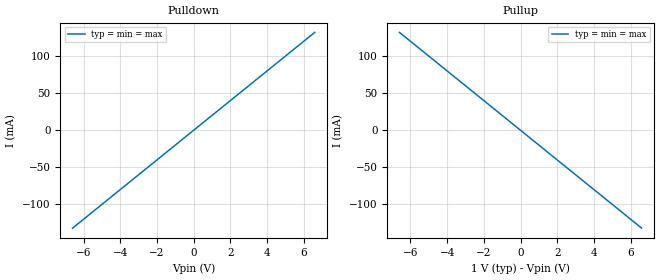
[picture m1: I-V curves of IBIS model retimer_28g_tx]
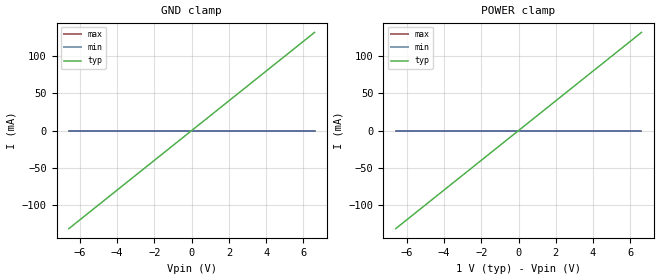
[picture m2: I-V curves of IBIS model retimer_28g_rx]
[IBIS Ver]   6.0
[File Name]   retimer_28g.ibs
[File Rev]   4
[Component]   retimer_28g
[Manufacturer] Texas Instruments, Inc.
[Package]
R_pkg  0.0   NA   NA
L_pkg  0.0   NA   NA
C_pkg  0.0   NA   NA
[Pin]   signal_name   model_name   R_pin L_pin  C_pin
1p   retimer_28g_rx_1p   retimer_28g_rx
1n   retimer_28g_rx_1n   retimer_28g_rx
2p   retimer_28g_tx_2p   retimer_28g_tx
2n   retimer_28g_tx_2n   retimer_28g_tx
[Diff_Pin] inv_pin vdiff tdelay_typ tdelay_min tdelay_max
1p   1n   NA   NA   NA   NA
2p   2n   NA   NA   NA   NA
[Repeater Pin] tx_non_inv_pin
1p 2p
| Models and submodels in the file (2): retimer_28g_tx (Output), retimer_28g_rx (Input)
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[Model] retimer_28g_tx
Model_type Output
C_comp 0p 0p 0p
Cref = 0
Vref = 0.5
Rref = 50
Vmeas = 0.5
[Temperature_Range] 25 125 0
[Voltage Range] 1.0 1.0 1.0
[Algorithmic Model]
Executable Windows_cl16.00.40219.01_64 retimer_28g_tx_x64_12_2015.dll retimer_28g_tx_08_2017.ami
Executable Windows_cl16.00.40219.01_32 retimer_28g_tx_12_2015.dll retimer_28g_tx_08_2017.ami
[End Algorithmic Model]
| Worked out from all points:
|   slope of the pulldown table from 0 to 0.15 V, typ, clamps not added: 50 ohm
|   slope of the pullup table from 0 to 0.15 V, typ, clamps not added: 50 ohm
[Pulldown]
-6.6V     -132mA     -132mA     -132mA
0V        0A         0A         0A
6.6V      132mA      132mA      132mA
[Pullup]
-6.6V     132mA      132mA      132mA
0V        0A         0A         0A
6.6V      -132mA     -132mA     -132mA
[GND Clamp]
-6.6V     0A         0A         0A
0V        0A         0A         0A
6.6V      0A         0A         0A
[Power Clamp]
-6.6V     0A         0A         0A
0V        0A         0A         0A
6.6V      0A         0A         0A
[Ramp]
dV/dt_r 0.3/1.5p 0.3/1.5p 0.3/1.5p
dV/dt_f 0.3/1.5p 0.3/1.5p 0.3/1.5p
[Model] retimer_28g_rx
Model_type Input
C_comp 0p 0p 0p
Vinh = 0.25
Vinl = -0.25
[Temperature_Range] 25 125 0
[Voltage Range] 1.0 1.0 1.0
[Algorithmic Model]
Executable Windows_cl16.00.40219.01_64 retimer_28g_rx_x64_12_2015.dll retimer_28g_rx_08_2017.ami
Executable Windows_cl16.00.40219.01_32 retimer_28g_rx_12_2015.dll retimer_28g_rx_08_2017.ami
[End Algorithmic Model]
[GND Clamp]
-6.6V     -132mA     0A         0A
0V        0A         0A         0A
6.6V      132mA      0A         0A
[Power Clamp]
-6.6V     -132mA     0A         0A
0V        0A         0A         0A
6.6V      132mA      0A         0A
